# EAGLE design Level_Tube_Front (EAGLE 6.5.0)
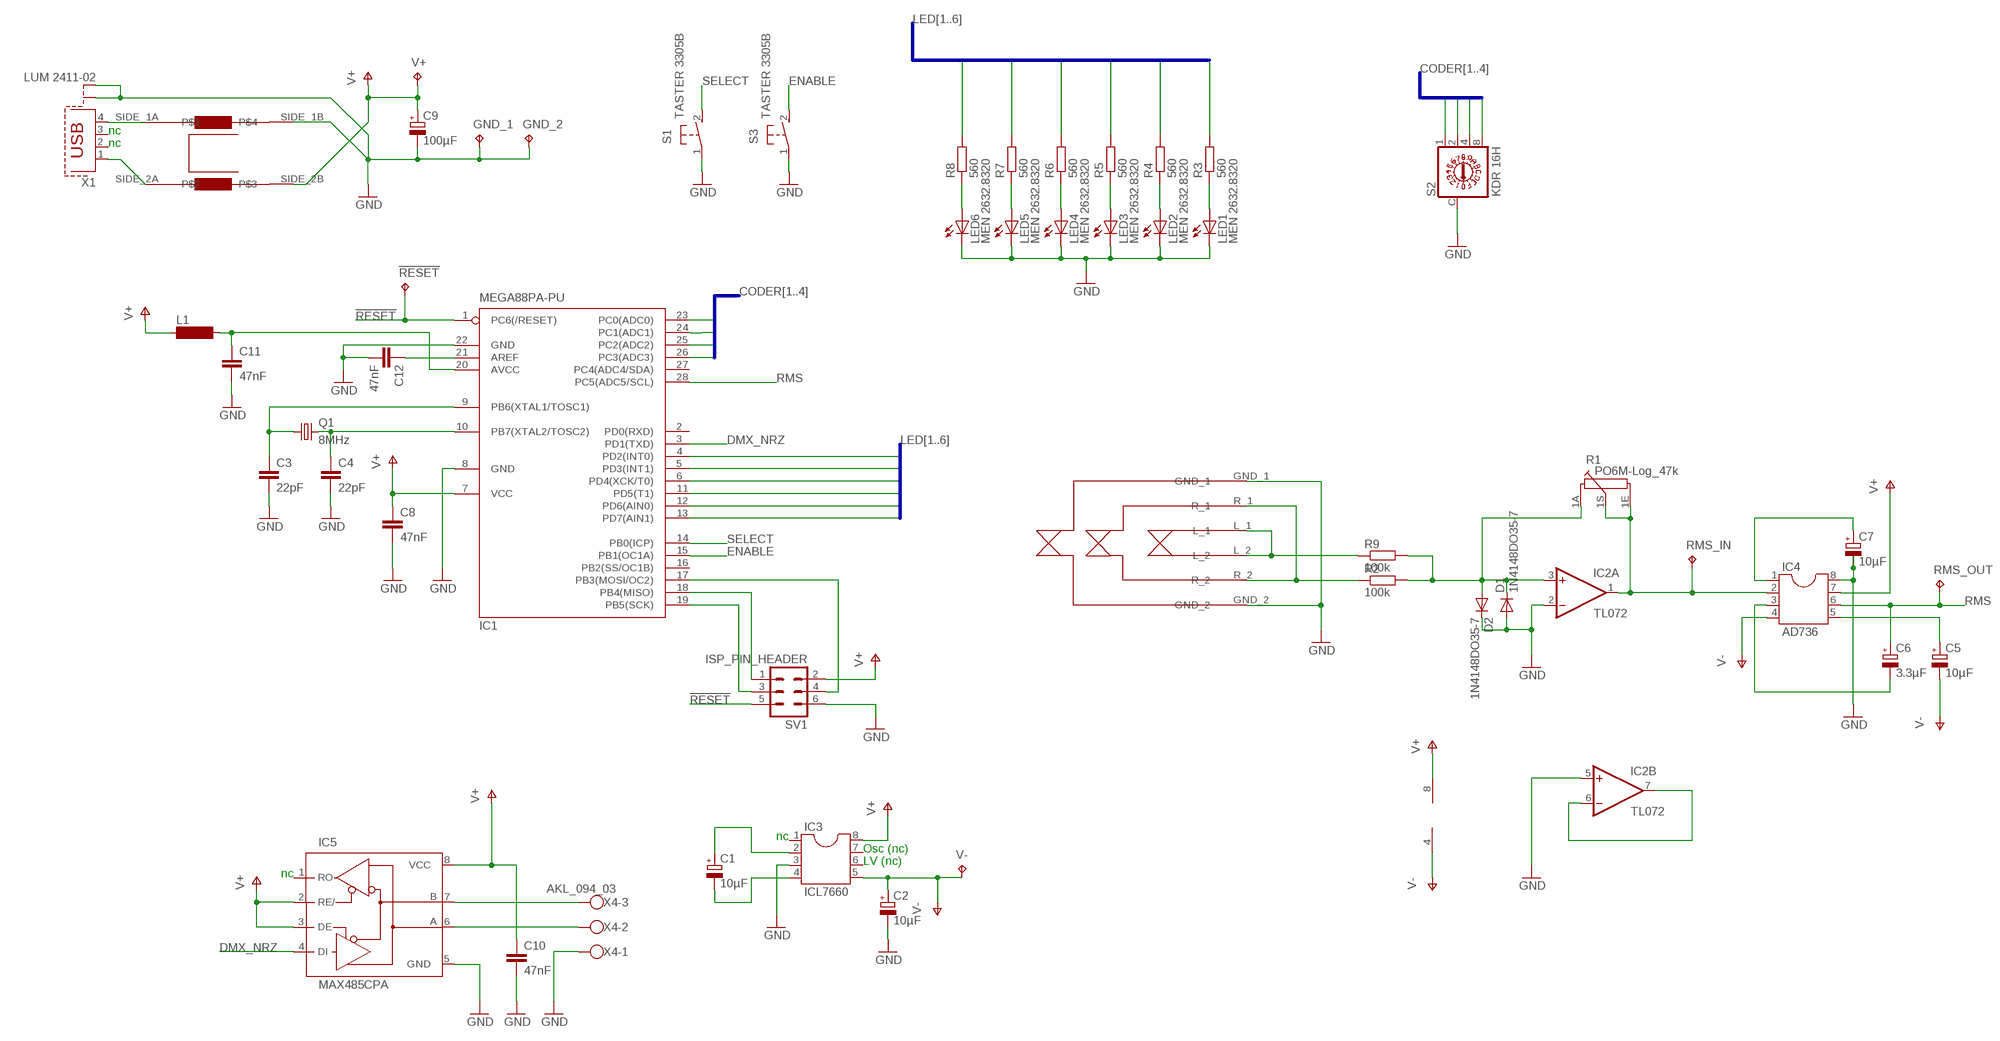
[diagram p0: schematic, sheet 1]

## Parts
!RESET  TPPAD1-13  [P1-13]
C1  10µF  CPOL-EUE2-5  [E2-5]
C2  10µF  CPOL-EUE2-5  [E2-5]
C3  22pF  C-EUC0805  [C0805]
C4  22pF  C-EUC0805  [C0805]
C5  10µF  CPOL-EUE2-5  [E2-5]
C6  3.3µF  CPOL-EUE2-5  [E2-5]
C7  10µF  CPOL-EUE2-5  [E2-5]
C8  47nF  C-EUC1206  [C1206]
C9  100µF  CPOL-EUE2-5  [E2-5]
C10  47nF  C-EUC1206  [C1206]
C11  47nF  C-EUC1206  [C1206]
C12  47nF  C-EUC1206  [C1206]
D1  1N4148DO35-7  [DO35-7]
D2  1N4148DO35-7  [DO35-7]
GND_1  TPPAD1-13  [P1-13]
GND_2  TPPAD1-13  [P1-13]
IC1  MEGA88PA-PU  MEGA8-P  [DIL28-3]
IC2  TL072  OPA2743PA  [DIL08]
IC3  ICL7660  DIL8  [DIL08]
IC4  AD736  DIL8  [DIL08]
IC5  MAX485CPA  MAX3468CPA  [DIL08]
L1  SM-1206  [SM-1206]
LED1  MEN 2632.8320  TLLR4400  [LED3MM]
LED2  MEN 2632.8320  TLLR4400  [LED3MM]
LED3  MEN 2632.8320  TLLR4400  [LED3MM]
LED4  MEN 2632.8320  TLLR4400  [LED3MM]
LED5  MEN 2632.8320  TLLR4400  [LED3MM]
LED6  MEN 2632.8320  TLLR4400  [LED3MM]
Q1  8MHz  CRYSTALHC49S  [HC49/S]
R1  PO6M-Log_47k  PC16S  [PC16S]
R2  100k  R-EU_0207/7  [0207/7]
R3  560  R-EU_M1206  [M1206]
R4  560  R-EU_M1206  [M1206]
R5  560  R-EU_M1206  [M1206]
R6  560  R-EU_M1206  [M1206]
R7  560  R-EU_M1206  [M1206]
R8  560  R-EU_M1206  [M1206]
R9  100k  R-EU_0207/7  [0207/7]
RMS_IN  TPPAD1-13  [P1-13]
RMS_OUT  TPPAD1-13  [P1-13]
S1  TASTER 3305B  31-XX  [B3F-31XX]
S2  KDR 16H  P103L  [P101L]
S3  TASTER 3305B  31-XX  [B3F-31XX]
SV1  ISP_PIN_HEADER  MA03-2  [MA03-2]
U$1  KLINKENBUCHSE_6.35_NR-J6HF  KLINKENBUCHSE_6.35  [STANDARD]
U$2  COMMON_MODE_CHOKE_CAF 0,5-47  COMMON_MODE_CHOKE  [COMMON_MODE]
V+  TPPAD1-13  [P1-13]
V-  TPPAD1-13  [P1-13]
X1  LUM 2411-02  PN61729-S  [PN61729-S]
X4  AKL_094_03  W237-103  [W237-103]

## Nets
!RESET: !RESET.TP IC1.1(PC6(/RESET)) SV1.5
AVCC: C11.1 IC1.20(AVCC) L1.2
CODER1: IC1.23(PC0(ADC0)) S2.1
CODER2: IC1.24(PC1(ADC1)) S2.2
CODER3: IC1.25(PC2(ADC2)) S2.4
CODER4: IC1.26(PC3(ADC3)) S2.8
DMX_NRZ: IC1.3(PD1(TXD)) IC5.4(DI)
ENABLE: IC1.15(PB1(OC1A)) S3.2(S)
GND: C2.- C3.2 C4.2 C7.- C8.2 C9.- C10.2 C11.2 C12.2 D1.A D2.C GND_1.TP GND_2.TP IC1.8(GND) IC1.22(GND) IC2.2(A:-IN) IC2.5(B:+IN) IC3.3 IC4.8 IC5.5(GND) LED1.K(C) LED2.K(C) LED3.K(C) LED4.K(C) LED5.K(C) LED6.K(C) S1.1(P) S2.C S3.1(P) SV1.6 U$1.GND_1 U$1.GND_2 U$2.SIDE_1B X1.S1 X1.S2 X4.1
LED1: IC1.13(PD7(AIN1)) R3.2
LED2: IC1.12(PD6(AIN0)) R4.2
LED3: IC1.11(PD5(T1)) R5.2
LED4: IC1.6(PD4(XCK/T0)) R6.2
LED5: IC1.5(PD3(INT1)) R7.2
LED6: IC1.4(PD2(INT0)) R8.2
N$1: IC1.17(PB3(MOSI/OC2)) SV1.4
N$2: R9.1 U$1.L_1 U$1.L_2
N$3: R2.1 U$1.R_1 U$1.R_2
N$4: IC1.18(PB4(MISO)) SV1.1
N$5: LED6.A R8.1
N$6: LED5.A R7.1
N$7: LED4.A R6.1
N$8: LED3.A R5.1
N$9: LED2.A R4.1
N$10: LED1.A R3.1
N$11: IC1.19(PB5(SCK)) SV1.3
N$12: U$2.SIDE_1A X1.4
N$13: C1.- IC3.4
N$14: C1.+ IC3.2
N$15: C3.1 IC1.9(PB6(XTAL1/TOSC1)) Q1.1
N$16: C4.1 IC1.10(PB7(XTAL2/TOSC2)) Q1.2
N$17: IC2.1(A:OUT) IC4.2 R1.1E R1.1S RMS_IN.TP
N$18: C5.+ IC4.5
N$19: IC2.6(B:-IN) IC2.7(B:OUT)
N$20: C6.- IC4.3
N$21: C7.+ IC4.1
N$22: IC5.7(B) X4.3
N$23: D1.C D2.A IC2.3(A:+IN) R1.1A R2.2 R9.2
N$24: IC5.6(A) X4.2
N$25: C12.1 IC1.21(AREF)
N$27: U$2.SIDE_2A X1.1
RMS: C6.+ IC1.28(PC5(ADC5/SCL)) IC4.6 RMS_OUT.TP
SELECT: IC1.14(PB0(ICP)) S1.2(S)
V+: C8.1 C9.+ C10.1 IC1.7(VCC) IC2.8(P:V+) IC3.8 IC4.7 IC5.2(RE/) IC5.3(DE) IC5.8(VCC) L1.1 SV1.2 U$2.SIDE_2B V+.TP
V-: C2.+ C5.- IC2.4(P:V-) IC3.5 IC4.4 V-.TP
Unconnected: IC1.2(PD0(RXD)) IC1.16(PB2(SS/OC1B)) IC1.27(PC4(ADC4/SDA)) IC3.1 IC3.6 IC3.7 IC5.1(RO) X1.2 X1.3

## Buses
LED[1..6]
CODER[1..4]

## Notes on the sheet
- nc
- nc
- nc
- Osc (nc)
- LV (nc)
- nc

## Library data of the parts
!RESET GND_1 GND_2 RMS_IN RMS_OUT V+ V- = testpad:TP: Test pad
C1 C2 C5-C7 C9 = rcl:CPOL-EU: POLARIZED CAPACITOR, European symbol
C3 C4 C8 C10-C12 = rcl:C-EU: CAPACITOR, European symbol
D1 D2 = diode:1N4148: DIODE
IC1 = atmel:MEGA8-P: MICROCONTROLLER 8 Kbytes FLASH, 1 kbytes SRAM, 512 bytes EEPROM, USART, 4-channel 10 bit ADC, 2-channel 8 bit ADC Pin compatible with Atmega48, ATMega88, ATMega168 Source: avr.lbr; OC_FARNELL: unknown; OC_NEWARK: unknown
IC2 = linear:OPA2743: 12V, 7MHz, CMOS, Rail-to-Rail I/O Dual OP AMP Source: http://focus.ti.com/lit/ds/sbos201/sbos201.pdf
IC3 IC4 = ic-package:DIL8: Dual In Line / Socket
IC5 = maxim:MAX34*: +5V, Fail-Safe, 40Mbps, Profibus RS-485/RS-422 Transceivers Source: MAX3465-MAX3469.pdf; OC_FARNELL: unknown; OC_NEWARK: unknown
L1 = inductor-neosid:SM-1206: INDUCTOR; OC_FARNELL: unknown; OC_NEWARK: unknown
LED1-LED6 = led:TLLR4400: Low Current (2mA) LED 3 mm Tinted Diffused Package color RED; MF: VISHAY SEMICONDUCTOR; OC_FARNELL: 1612437
Q1 = crystal:CRYSTAL: CRYSTAL; OC_FARNELL: 1667008; OC_NEWARK: unknown
R1 = piher:PC16S: POTENTIOMETER single carbon potentiometer, 16 mm, S3ROH; OC_FARNELL: 4452940; OC_NEWARK: unknown
R2-R9 = rcl:R-EU_: RESISTOR, European symbol
S1 S3 = switch-omron:31-XX: OMRON SWITCH; MPN: B3F-3100; OC_FARNELL: 959704; OC_NEWARK: 36M3582
S2 = switch-dil:P103L: DIL/CODE SWITCH; OC_FARNELL: unknown; OC_NEWARK: unknown
SV1 = con-lstb:MA03-2: PIN HEADER; OC_FARNELL: unknown; OC_NEWARK: unknown
U$1 = leveltube:KLINKENBUCHSE_6.35: Klinkenbuchse für 6.35 mm Neutronik NEUTRIK NR-J6HF
U$2 = leveltube:COMMON_MODE_CHOKE
X1 = con-berg:PN61729-S: BERG USB connector; OC_FARNELL: unknown; OC_NEWARK: unknown
X4 = con-wago-500:W237-103: WAGO SCREW CLAMP; MPN: 237-103; OC_FARNELL: unknown; OC_NEWARK: 18M7116

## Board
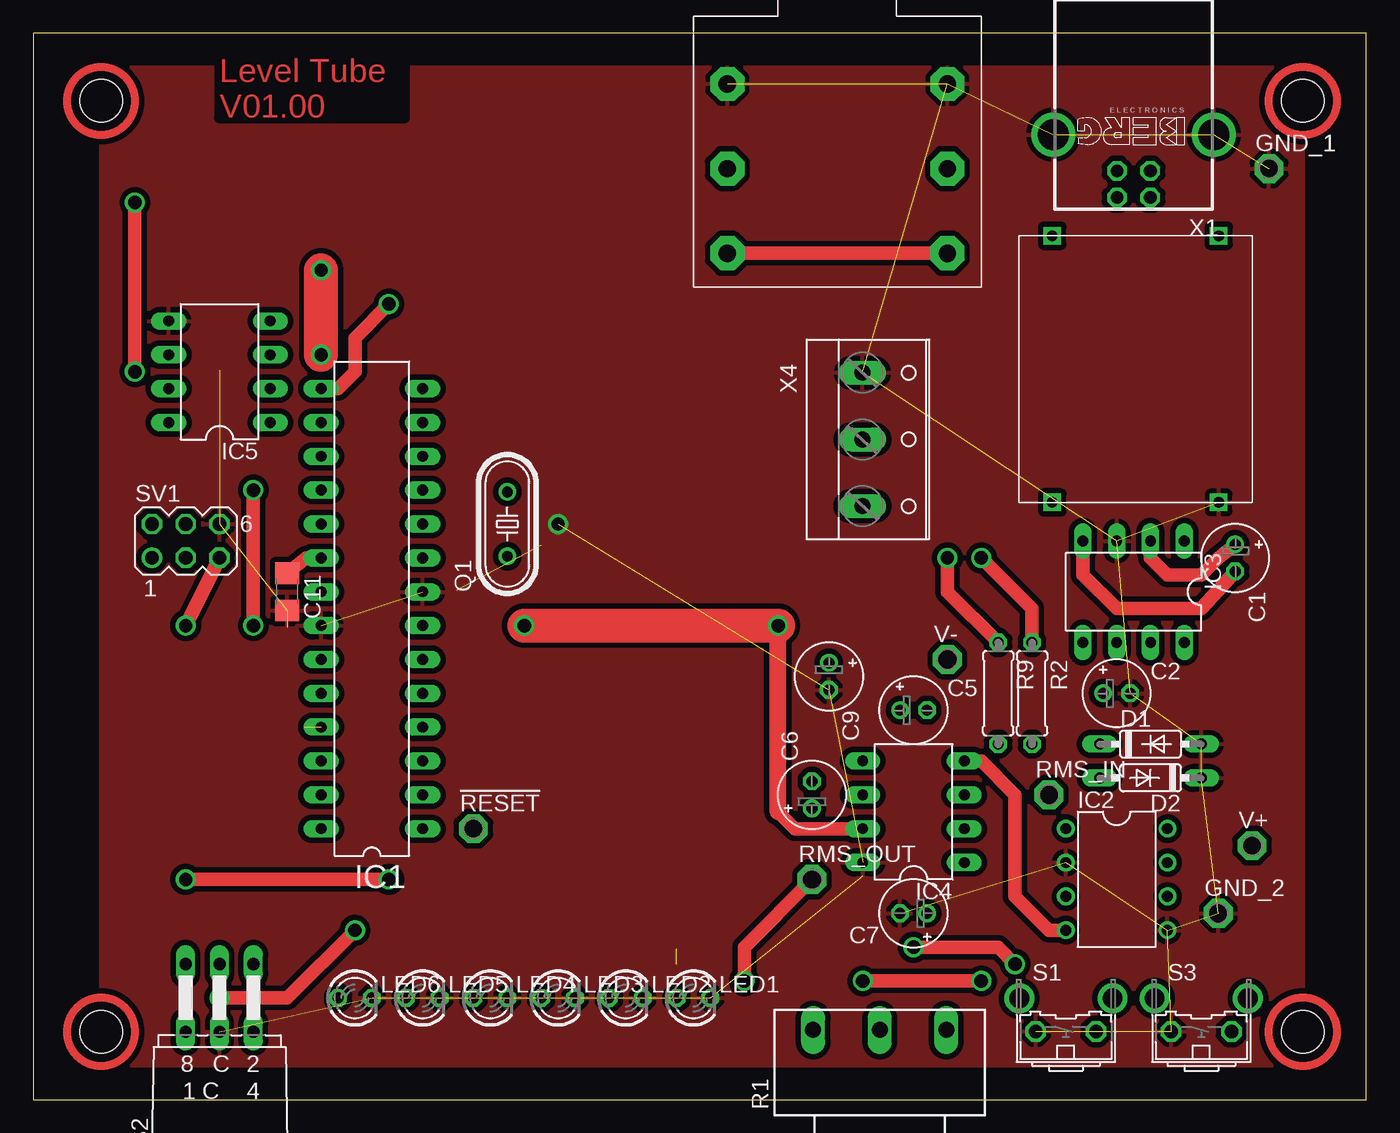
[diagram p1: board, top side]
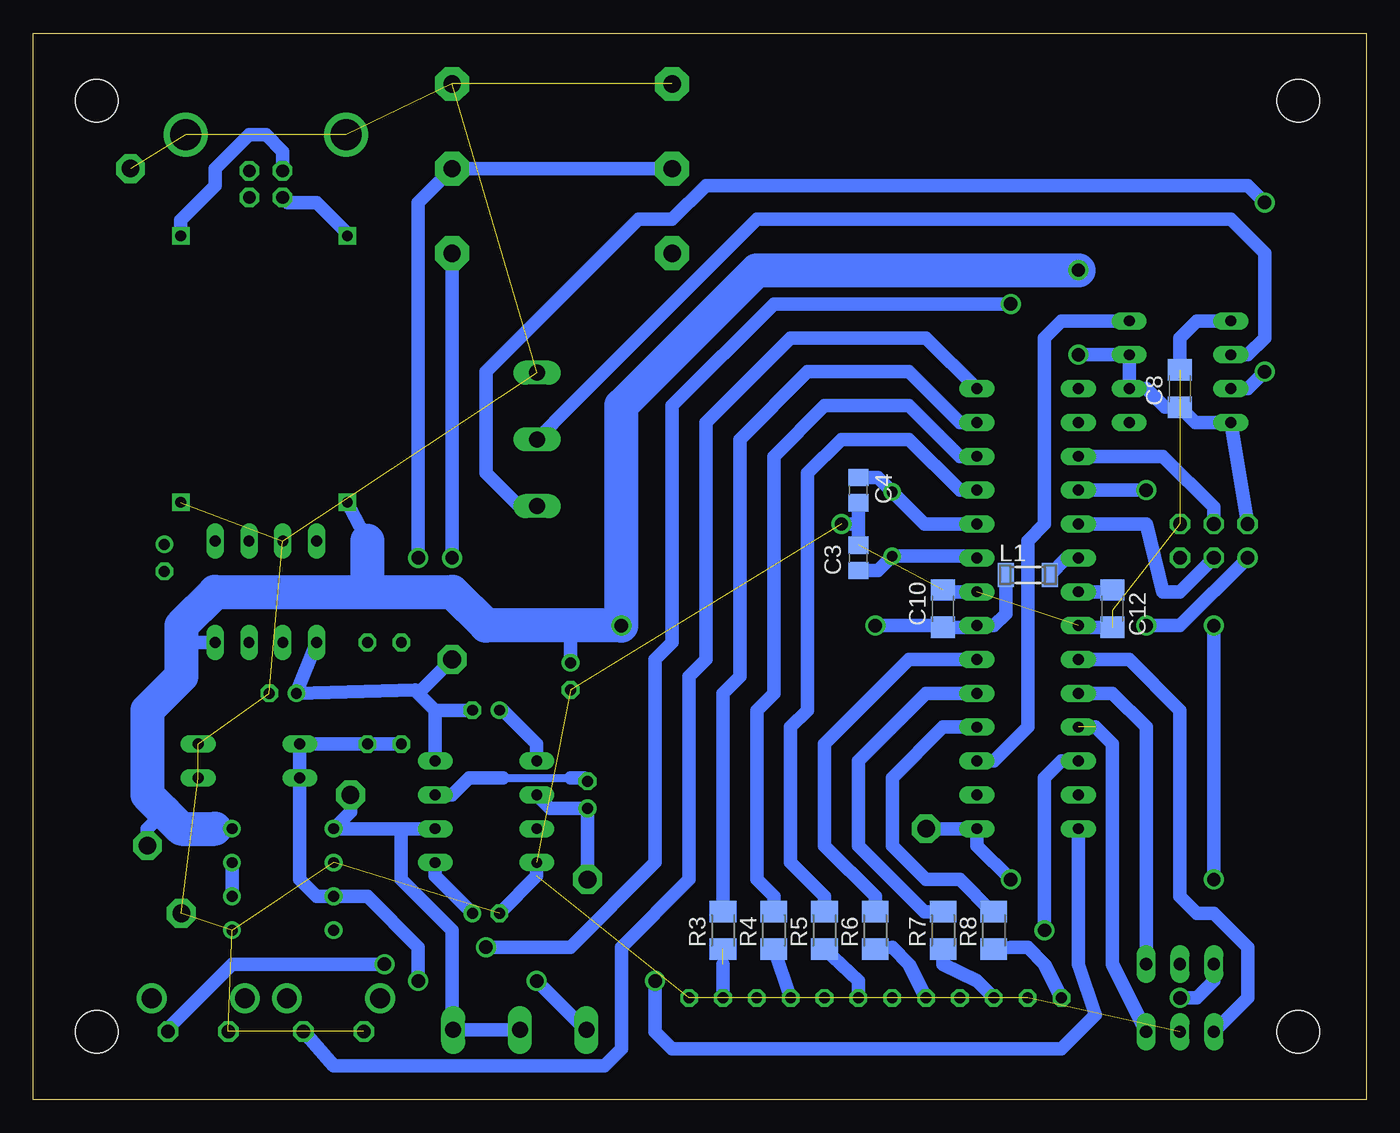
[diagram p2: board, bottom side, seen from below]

Size 100 x 80 mm. Coordinates in mm from the lower left corner, seen from the top.
Outline: 0,0 100,0 100,80 0,80 0,0
Copper layers (1*16): Top 0.035mm / dielectric 1.5mm / Bottom 0.035mm
Design rules "default *": minimum track width 10mil, minimum drill 24mil, track to track 12mil, track to pad 12mil, pad to pad 12mil, via to via 12mil, smd to smd 12mil, copper to edge 40mil, drill to drill 12mil, minimum pad ring 10mil, minimum via ring 8mil, stop-mask expansion 4mil, vias tented up to drill 0mil, thermal gap 15mil
Holes 3.2 mm at 5.08,74.93 5.08,5.08 95.25,5.08 95.25,74.93

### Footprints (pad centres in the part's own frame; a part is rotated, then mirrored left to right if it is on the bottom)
P1-13 = drill 1.321 pad 2.159 octagon: TP 0,0
E2-5 = drill 0.813 pad 1.27: + -1.016,0 | drill 0.813 pad 1.27 octagon: - 1.016,0
C0805 = smd 1.3 x 1.5: 1 -0.95,0; 2 0.95,0
C1206 = smd 1.6 x 1.8: 1 -1.4,0; 2 1.4,0
DO35-7 = drill 0.813 long: A 3.81,0; C -3.81,0
DIL28-3 = drill 0.813 long: 1 -16.51,-3.81; 2 -13.97,-3.81; 3 -11.43,-3.81; 4 -8.89,-3.81; 5 -6.35,-3.81; 6 -3.81,-3.81; 7 -1.27,-3.81; 8 1.27,-3.81; 9 3.81,-3.81; 10 6.35,-3.81; 11 8.89,-3.81; 12 11.43,-3.81; 13 13.97,-3.81; 14 16.51,-3.81; 15 16.51,3.81; 16 13.97,3.81; 17 11.43,3.81; 18 8.89,3.81; 19 6.35,3.81; 20 3.81,3.81; 21 1.27,3.81; 22 -1.27,3.81; 23 -3.81,3.81; 24 -6.35,3.81; 25 -8.89,3.81; 26 -11.43,3.81; 27 -13.97,3.81; 28 -16.51,3.81
DIL08 = drill 0.813 pad 1.27: 1 -3.81,-3.81; 2 -1.27,-3.81; 3 1.27,-3.81; 4 3.81,-3.81; 5 3.81,3.81; 6 1.27,3.81; 7 -1.27,3.81; 8 -3.81,3.81
DIL08' = drill 0.813 long: 1 -3.81,-3.81; 2 -1.27,-3.81; 3 1.27,-3.81; 4 3.81,-3.81; 5 3.81,3.81; 6 1.27,3.81; 7 -1.27,3.81; 8 -3.81,3.81
SM-1206 = smd 1.2 x 1.8: 1 -1.65,0; 2 1.65,0
LED3MM = drill 0.813 octagon: A -1.27,0; K 1.27,0
HC49/S = drill 0.813: 1 -2.413,0; 2 2.413,0
PC16S = drill 1.2 long: 1A -5,6.5; 1E 5,6.5; 1S 0,6.5
0207/7 = drill 0.813 octagon: 1 -3.81,0; 2 3.81,0
M1206 = smd 1.6 x 2: 1 -1.4,0; 2 1.4,0
B3F-31XX = drill 1.016 octagon: 1 -2.261,-1.245; 2 2.261,-1.245 | drill 1.499 pad 2.159: 3 -3.505,1.245; 4 3.505,1.245
P101L = drill 0.914 long: 1 -2.54,2.54; 2 2.54,7.62; 4 2.54,2.54; 8 -2.54,7.62; C 0,2.54; C1 0,7.62
MA03-2 = drill 1.016: 1 -2.54,-1.27 | drill 1.016 octagon: 2 -2.54,1.27; 3 0,-1.27; 4 0,1.27; 5 2.54,-1.27; 6 2.54,1.27
STANDARD = drill 1.3 pad 2.54 octagon: GND_1 2.54,15.24; GND_2 19.05,15.24; L_1 2.54,2.54; L_2 19.05,2.54; R_1 2.54,8.89; R_2 19.05,8.89
COMMON_MODE = drill 0.8 square: SIDE_1A 2.5,2.5; SIDE_1B 2.5,22.5; SIDE_2A 15,2.5; SIDE_2B 15,22.5
PN61729-S = drill 0.95 octagon: 1 1.25,4.71; 2 -1.25,4.71; 3 -1.25,2.71; 4 1.25,2.71 | drill 2.3 pad 2.9: S1 -6.02,0; S2 6.02,0
W237-103 = drill 1.194 long: 1 -5,-1.29; 2 0,-1.29; 3 5,-1.29

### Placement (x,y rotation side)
!RESET  33.02,20.32 0 top
C1  90.17,40.64 270 top
C2  81.28,30.48 0 top
C3  38.1,40.64 90 bottom
C4  38.1,45.72 270 bottom
C5  66.04,29.21 0 top
C6  58.42,22.86 90 top
C7  66.04,13.97 180 top
C8  13.97,53.34 90 bottom
C9  59.69,31.75 270 top
C10  31.75,36.83 90 bottom
C11  19.05,38.1 270 top
C12  19.05,36.83 270 bottom
D1  83.82,26.67 0 top
D2  83.82,24.13 180 top
GND_1  92.71,69.85 0 top
GND_2  88.9,13.97 0 top
IC1  25.4,36.83 90 top
IC2  81.28,16.51 270 top
IC3  ICL7660  [DIL08']  82.55,38.1 180 top
IC4  AD736  [DIL08']  66.04,21.59 90 top
IC5  MAX485CPA  [DIL08']  13.97,54.61 90 top
L1  25.4,39.37 0 bottom
LED1  49.53,7.62 0 top
LED2  44.45,7.62 0 top
LED3  39.37,7.62 0 top
LED4  34.29,7.62 0 top
LED5  29.21,7.62 0 top
LED6  24.13,7.62 0 top
Q1  35.56,43.18 90 top
R1  63.5,-1.27 0 top
R2  74.93,30.48 270 top
R3  48.26,12.7 90 bottom
R4  44.45,12.7 90 bottom
R5  40.64,12.7 90 bottom
R6  36.83,12.7 90 bottom
R7  31.75,12.7 90 bottom
R8  27.94,12.7 90 bottom
R9  72.39,30.48 270 top
RMS_IN  76.2,22.86 0 top
RMS_OUT  58.42,16.51 0 top
S1  77.47,6.35 0 top
S2  13.97,2.54 0 top
S3  87.63,6.35 0 top
SV1  11.43,41.91 0 top
U$1  49.53,60.96 0 top
U$2  91.44,67.31 180 top
V+  91.44,19.05 0 top
V-  68.58,33.02 0 top
X1  82.55,72.39 180 top
X4  63.5,49.53 270 top

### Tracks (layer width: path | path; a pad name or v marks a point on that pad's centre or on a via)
!RESET  (via drill 1)
  Top 1.016: SV1.5 v11.43,35.56 | v11.43,16.51 v26.67,16.51
  Bottom 1.016: !RESET.TP IC1.1 29.21,19.05 v26.67,16.51 | v11.43,16.51 v11.43,35.56
AVCC
  Top 1.016: C11.1 20.45,40.64 IC1.20
  Bottom 1.016: 21.46,40.77 IC1.20 22.48,40.64 L1.2
CODER1
  Bottom 1.016: S2.1 8.89,7.62 8.89,11.43 11.43,13.97 12.7,13.97 13.97,15.24 13.97,29.21 17.78,33.02 IC1.23
CODER2
  Bottom 1.016: S2.2 16.51,27.94 19.05,30.48 IC1.24
CODER3  (1 unrouted)
  Bottom 1.016: S2.4 19.05,10.16 19.05,26.67 20.32,27.94
CODER4  (via drill 1)
  Top 1.016: v13.97,7.62 19.05,7.62 v24.13,12.7
  Bottom 1.016: S2.8 11.43,8.89 12.7,7.62 v13.97,7.62 | v24.13,12.7 24.13,24.13 22.86,25.4 IC1.26
DMX_NRZ
  Bottom 1.016: IC1.3 27.94,25.4 25.4,27.94 25.4,41.91 24.13,43.18 24.13,57.15 22.86,58.42 IC5.4
ENABLE  (via drill 1)
  Top 1.016: IC1.15 22.86,53.34 24.13,54.61 24.13,57.15 v26.67,59.69 | v73.66,10.16 72.39,11.43 v66.04,11.43
  Bottom 1.016: v26.67,59.69 44.45,59.69 52.07,52.07 52.07,34.29 53.34,33.02 53.34,17.78 59.69,11.43 v66.04,11.43 | S3.2 89.89,5.36 85.09,10.16 v73.66,10.16
GND  (via drill 1)  (30 unrouted)
  Bottom 1.016: IC1.22 21.46,35.43 C12.2 | C8.2 13.97,57.15 12.7,58.42 IC5.5 | IC1.8 31.62,38.1 C10.2 | C7.- 62.23,16.76 IC4.8 | 38.1,43.18 C4.2 | C3.2 38.1,43.18 | 38.1,43.18 v39.37,43.18
  pour Top (isolate 0.406): 5.08,77.47 95.25,77.47 95.25,2.54 5.08,2.54
LED1
  Bottom 1.016: IC1.13 30.48,50.8 34.29,54.61 41.91,54.61 46.99,49.53 46.99,31.75 48.26,30.48 R3.2
LED2
  Bottom 1.016: R4.2 44.45,15.24 45.72,16.51 45.72,29.21 44.45,30.48 44.45,48.26 40.64,52.07 34.29,52.07 30.48,48.26 IC1.12
LED3
  Bottom 1.016: IC1.11 30.48,45.72 34.29,49.53 39.37,49.53 41.91,46.99 41.91,29.21 43.18,27.94 43.18,17.78 40.64,15.24 R5.2
LED4
  Bottom 1.016: R6.2 36.83,15.24 40.64,19.05 40.64,26.67 34.29,33.02 IC1.6
LED5
  Bottom 1.016: R7.2 33.15,14.1 38.1,19.05 38.1,25.4 33.02,30.48 IC1.5
LED6
  Bottom 1.016: R8.2 28.07,14.1 30.48,16.51 33.02,16.51 35.56,19.05 35.56,24.13 31.75,27.94 IC1.4
N$1
  Bottom 1.016: SV1.4 11.43,44.45 15.24,48.26 IC1.17
N$2  (via drill 1)
  Top 1.016: R9.1 68.58,38.1 v68.58,40.64 | U$1.L_1 U$1.L_2
  Bottom 1.016: v68.58,40.64 U$1.L_2
N$3  (via drill 1)
  Top 1.016: v71.12,40.64 74.93,36.83 R2.1
  Bottom 1.016: U$1.R_1 U$1.R_2 71.12,67.31 v71.12,40.64
N$4  (via drill 1)
  Top 1.016: v16.51,35.56 v16.51,45.72
  Bottom 1.016: SV1.1 13.97,35.56 v16.51,35.56 | IC1.18 v16.51,45.72
N$5
  Bottom 1.016: R8.1 26.67,11.43 25.4,11.43 24.13,10.16 LED6.A
N$6
  Bottom 1.016: R7.1 31.75,10.16 29.21,8.89 LED5.A
N$7
  Bottom 1.016: R6.1 35.56,11.43 34.29,10.16 LED4.A
N$8
  Bottom 1.016: R5.1 38.1,8.89 LED3.A
N$9
  Bottom 1.016: R4.1 LED2.A
N$10  (1 unrouted)
  Bottom 1.016: LED1.A 48.26,10.16
N$11
  Bottom 1.016: IC1.19 16.51,43.18 15.24,38.1 13.97,38.1 SV1.3
N$12
  Bottom 1.016: U$2.SIDE_1A 88.94,66 86.36,68.58 86.36,69.85 83.82,72.39 82.55,72.39 81.28,71.12 81.28,69.7 X1.4
N$13
  Top 1.016: C1.- 87.63,36.83 81.28,36.83 78.74,39.37 IC3.4
N$14
  Top 1.016: C1.+ 88.9,40.64 87.63,39.37 85.09,39.37 83.82,40.64 IC3.2
N$15
  Bottom 1.016: C3.1 36.64,39.69 Q1.1 29.34,40.77 IC1.9
N$16
  Bottom 1.016: C4.1 36.64,46.67 Q1.2 33.15,43.18 IC1.10
N$17
  Bottom 1.016: 72.39,20.32 IC2.1 76.2,21.59 RMS_IN.TP | 72.39,20.32 IC4.2 | R1.1E R1.1S 68.58,5.23 68.58,12.7 72.39,16.51 72.39,20.32
N$18
  Bottom 1.016: IC4.5 62.23,26.67 64.77,29.21 C5.+
N$19
  Bottom 1.016: IC2.6 IC2.7
N$20
  Bottom 0.61: 64.77,24.13 59.69,24.13
  Bottom 1.016: C6.- 58.67,24.13 59.69,24.13 | IC4.3 68.58,22.86 67.31,24.13 64.77,24.13
N$21
  Bottom 1.016: C7.+ 69.85,16.76 IC4.1
N$22  (via drill 1)
  Top 1.016: v7.62,54.61 v7.62,67.31
  Bottom 1.016: IC5.7 8.89,53.34 v7.62,54.61 | v7.62,67.31 8.89,68.58 49.53,68.58 52.07,66.04 54.61,66.04 66.04,54.61 66.04,46.99 63.5,44.45 63.5,44.51 X4.3
N$23  (via drill 1)
  Top 1.016: v62.23,8.89 v71.12,8.89
  Bottom 1.016: R9.2 R2.2 D1.C D2.A 80.01,16.51 78.74,15.24 IC2.3 74.93,15.24 71.12,11.43 v71.12,8.89 | R1.1A 58.5,5.16 v62.23,8.89
N$24
  Bottom 1.016: IC5.6 8.89,55.88 7.62,57.15 7.62,63.5 10.16,66.04 45.72,66.04 59.69,52.07 X4.2 63.5,49.53
N$25
  Bottom 1.016: C12.1 19.18,38.1 IC1.21
N$27
  Bottom 1.016: U$2.SIDE_2A 76.44,65.01 78.74,67.31 80.93,67.31 X1.1
RMS  (via drill 1)
  Top 1.016: v53.34,8.89 53.34,11.43 RMS_OUT.TP
  Bottom 1.016: IC1.28 21.59,10.16 20.32,6.35 22.86,3.81 52.07,3.81 53.34,5.08 v53.34,8.89 | IC4.6 61.21,21.84 C6.+ RMS_OUT.TP
SELECT
  Bottom 1.016: S1.2 77.47,2.54 57.15,2.54 55.88,3.81 55.88,11.43 50.8,16.51 50.8,31.75 49.53,33.02 49.53,50.8 43.18,57.15 33.02,57.15 IC1.14
V+  (via drill 1)
  Top 1.016: IC4.7 57.15,20.32 55.88,21.59
  Top 1.27: 55.88,21.59 v55.88,35.56
  Top 2.54: v36.83,35.56 v55.88,35.56 | v21.59,55.88 v21.59,62.23
  Bottom 1.016: L1.1 27.05,36.45 27.94,35.56 IC1.7 29.34,35.43 C10.1 31.75,35.56 v36.83,35.56 | SV1.2 IC5.8 12.83,50.8 C8.1 15.11,51.94 16.51,53.34 IC5.2 IC5.3 v21.59,55.88 | 86.36,20.32 IC2.8 | IC3.8 88.9,34.29 | V+.TP 91.44,20.32 90.17,21.59 | C9.+ 59.69,35.56 | 74.93,41.91 U$2.SIDE_2B
  Bottom 2.54: v21.59,62.23 45.72,62.23 55.88,52.07 v55.88,35.56 59.69,35.56 66.04,35.56 68.58,38.1 74.93,38.1 | 86.36,20.32 88.9,20.32 90.17,21.59 91.44,22.86 91.44,29.21 88.9,31.75 88.9,34.29 88.9,35.56 86.36,38.1 74.93,38.1 | 74.93,38.1 74.93,41.91
V-
  Top 1.016: IC2.4 76.2,12.7 73.66,15.24 73.66,22.86 71.12,25.4 IC4.4
  Bottom 1.016: 69.85,29.21 IC4.4 | 71.12,30.48 71.37,30.73 C2.+ IC3.5 | 71.12,30.48 69.85,29.21 | C5.- 69.85,29.21 | V-.TP 71.12,30.48
(copper drawn outside any net)
  shapes: Top circle x4

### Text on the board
Top: Level Tube / V01.00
